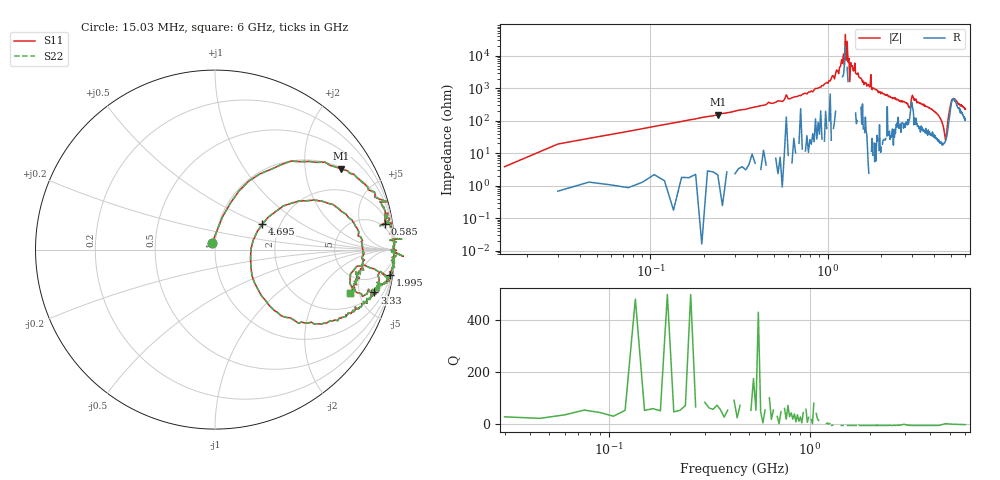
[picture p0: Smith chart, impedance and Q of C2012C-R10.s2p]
!	Network	Analyzer	HP8753E.07.74:	Oct	30	2002	Serial	No.	JP38451487
!	Hewlett-Packard
!	7	Sep	2009	12:12:40
!	Frequency	S11	S21	S12	S22
#	HZ	S	RI	R	50
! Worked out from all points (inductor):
!   400 points, 15.03 MHz to 6 GHz, reference 50 ohm
!   read as one part in series: L = 101 nH near 45.03 MHz
!   highest Q = 66.7 at 240 MHz (marker M1), where L = 103 nH
!   self-resonance near 1.23 GHz
!   S11 on the Smith chart (normalised r, x): 15.03 MHz: 0.96, +0.07; 585 MHz: 4, +12; 1.995 GHz: 1, -14; 3.33 GHz: 2.23, -6.84; 4.695 GHz: 1.62, +0.50; 6 GHz: 3.11, -4.06
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1.502992e7  -0.0168 0.0346  1.02 -0.0346  1.02 -0.0346  -0.0168 0.0346
3.002985e7  0.0415 0.182  0.959 -0.182  0.959 -0.182  0.0415 0.182
6.00297e7  0.133 0.326  0.867 -0.326  0.867 -0.326  0.133 0.326
2.400288e8  0.703 0.45  0.297 -0.45  0.297 -0.45  0.703 0.45
5.850271e8  0.947 0.142  0.053 -0.142  0.053 -0.142  0.947 0.142
1.020025e9  0.993 0.0569  0.0065 -0.0569  0.0065 -0.0569  0.993 0.0569
1.245024e9  0.982 -0.00296  0.0182 0.00296  0.0182 0.00296  0.982 -0.00296
1.260024e9  0.999 0.00198  0.000946 -0.00198  0.000946 -0.00198  0.999 0.00198
1.275024e9  1.01 -0.00458  -0.0129 0.00458  -0.0129 0.00458  1.01 -0.00458
1.290024e9  0.999 -0.00354  0.00058 0.00354  0.00058 0.00354  0.999 -0.00354
1.335023e9  1.05 -0.0378  -0.0536 0.0378  -0.0536 0.0378  1.05 -0.0378
1.350023e9  1 -0.0161  -0.00048 0.0161  -0.00048 0.0161  1 -0.0161
1.425023e9  1 -0.0165  -0.00293 0.0165  -0.00293 0.0165  1 -0.0165
1.605022e9  1 -0.0765  -0.00299 0.0765  -0.00299 0.0765  1 -0.0765
1.99502e9  0.977 -0.143  0.0232 0.143  0.0232 0.143  0.977 -0.143
2.01002e9  0.979 -0.132  0.0206 0.132  0.0206 0.132  0.979 -0.132
3.015015e9  0.917 -0.127  0.0834 0.127  0.0834 0.127  0.917 -0.127
3.330013e9  0.887 -0.239  0.113 0.239  0.113 0.239  0.887 -0.239
4.00501e9  0.757 -0.357  0.243 0.357  0.243 0.357  0.757 -0.357
4.695007e9  0.263 0.141  0.737 -0.141  0.737 -0.141  0.263 0.141
5.010005e9  0.81 0.0721  0.19 -0.0721  0.19 -0.0721  0.81 0.0721
6e9  0.754 -0.243  0.246 0.243  0.246 0.243  0.754 -0.243
